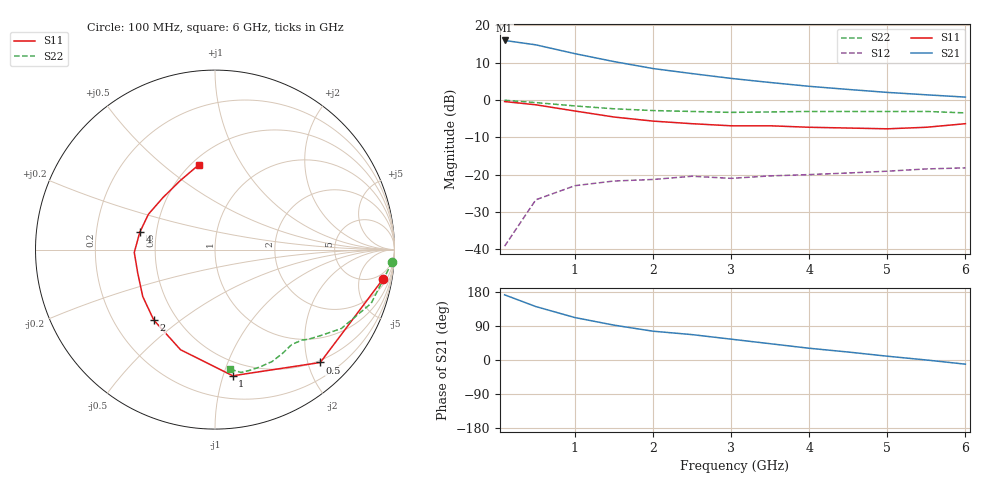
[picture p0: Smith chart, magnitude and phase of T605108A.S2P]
!AT-60510
!S-PARAMETERS at Vce=8V  Ic=2mA.  LAST UPDATED 07-21-92
# ghz s ma r 50
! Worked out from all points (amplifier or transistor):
!   13 points, 100 MHz to 6 GHz, reference 50 ohm
!   highest |S21| = 15.9 dB at 100 MHz (marker M1)
!   |S21| within 3 dB of that: start of sweep to 886.6 MHz
!   unconditionally stable (mu >= 1): 2.659 GHz to end of sweep
!   at 1 GHz: K = 0.42, MSG = 17.7 dB, |S12| = -23.0 dB
!   at 3 GHz: K = 1.20, MAG = 10.7 dB, |S12| = -21.0 dB
!   at 6 GHz: K = 1.33, MAG = 6.0 dB, |S12| = -18.2 dB
!   lowest NFmin = 1.40 dB at 1 GHz
!   S11 on the Smith chart (normalised r, x): 100 MHz: 3, -11; 500 MHz: 0.46, -2.22; 1 GHz: 0.38, -1.08; 2 GHz: 0.37, -0.40; 4 GHz: 0.40, +0.10; 6 GHz: 0.54, +0.67
0.1  0.95 -10.0  6.25 172.0  0.011 92.0  0.99 -4.0
0.5  0.86 -47.0  5.46 141.0  0.046 61.0  0.92 -19.0
1  0.71 -82.0  4.16 112.0  0.071 43.0  0.83 -32.0
1.5  0.59 -109.0  3.26 92.0  0.082 33.0  0.76 -39.0
2  0.52 -131.0  2.63 76.0  0.086 26.0  0.72 -44.0
2.5  0.48 -147.0  2.25 67.0  0.095 28.0  0.7 -46.0
3  0.45 -163.0  1.94 55.0  0.089 25.0  0.68 -51.0
3.5  0.45 -178.0  1.71 43.0  0.096 22.0  0.69 -57.0
4  0.43 167.0  1.52 31.0  0.1 23.0  0.7 -63.0
4.5  0.42 152.0  1.38 21.0  0.105 21.0  0.7 -69.0
5  0.41 135.0  1.26 10.0  0.111 18.0  0.7 -74.0
5.5  0.43 117.0  1.17 0.0  0.119 17.0  0.7 -78.0
6  0.48 101.0  1.09 -11.0  0.123 17.0  0.67 -83.0
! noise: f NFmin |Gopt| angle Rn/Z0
1  1.4  0.5  50  0.32
2  1.8  0.44  97  0.42
4  2.8  0.38  -163  0.42
